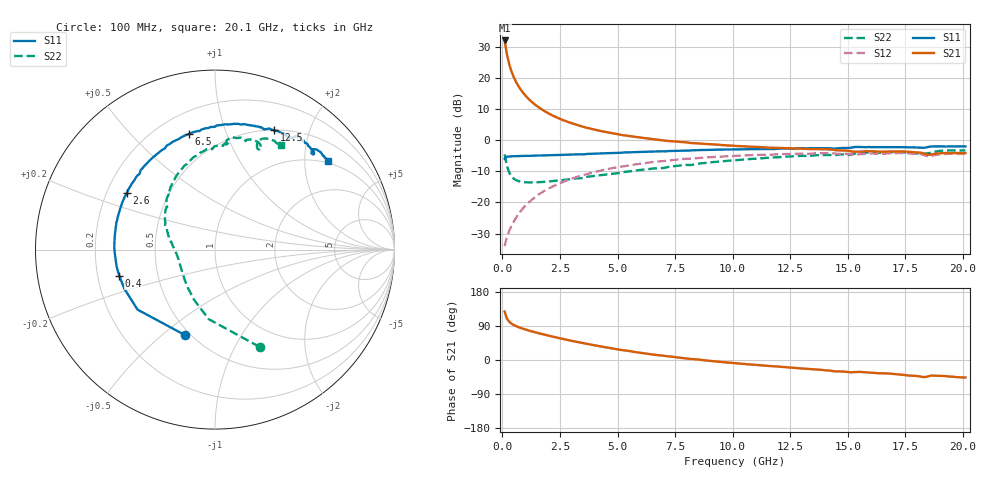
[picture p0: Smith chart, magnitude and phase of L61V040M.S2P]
!  Infineon Technologies AG
! BFR380L3 , PF131585-7, No.6, Th 09.10.01, soldered on pcb-board, measured with PP GSG850
!  Vce=1.0 V,  Ic=40.0 mA
! Common Emitter S-Parameters:  15. November 2001
#  GHz  S  MA  R  50
! f  S11  S21  S12  S22
! GHz  Mag  Ang  Mag  Ang  Mag  Ang  Mag  Ang
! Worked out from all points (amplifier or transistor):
!   201 points, 100 MHz to 20.1 GHz, reference 50 ohm
!   highest |S21| = 32.2 dB at 100 MHz (marker M1)
!   |S21| within 3 dB of that: start of sweep to 166.8 MHz
!   unconditionally stable (mu >= 1): 886.7 MHz to 4.66 GHz; 18.32 GHz to 18.54 GHz
!   at 3.4 GHz: K = 1.02, MAG = 7.1 dB, |S12| = -11.4 dB
!   at 10.1 GHz: K = 0.97, MSG = 1.6 dB, |S12| = -5.0 dB
!   at 20.1 GHz: K = 0.99, MSG = 0.1 dB, |S12| = -4.3 dB
!   S11 on the Smith chart (normalised r, x): 100 MHz: 0.47, -0.60; 400 MHz: 0.29, -0.12; 2.6 GHz: 0.28, +0.27; 6.5 GHz: 0.33, +0.75; 12.5 GHz: 0.50, +1.49; 20.1 GHz: 0.95, +2.58
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0.1  0.5047 -109.4  40.63 127.8  0.01979 59.6  0.5962 -65.4
0.2  0.546 -142.3  24.22 109.2  0.02799 54.9  0.389 -95.2
0.3  0.55 -156.6  16.86 101.1  0.0349 58.6  0.3032 -112.6
0.4  0.5532 -164.6  12.86 95.9  0.04201 61.6  0.2626 -124.7
0.5  0.5562 -170.0  10.37 92.2  0.04938 64.3  0.2413 -133.7
0.6  0.5566 -174.3  8.69 89.3  0.05715 65.7  0.2287 -140.5
0.7  0.5586 -177.6  7.484 86.7  0.06461 66.7  0.221 -146.0
0.8  0.561 179.3  6.567 84.5  0.0727 67.6  0.2162 -150.4
1  0.5624 174.5  5.288 80.5  0.08844 68.2  0.2116 -157.2
1.3  0.5655 168.5  4.101 75.2  0.1123 67.8  0.2105 -164.4
1.6  0.5697 162.9  3.362 70.3  0.136 66.6  0.2123 -169.6
2  0.5756 156.4  2.727 64.3  0.1668 64.4  0.2179 -175.1
2.6  0.5841 147.4  2.146 56.0  0.2119 60.5  0.2295 178.0
3.5  0.5955 135.0  1.657 44.5  0.2766 53.8  0.2474 169.5
4.9  0.6276 118.7  1.279 29.1  0.3642 43.2  0.2935 156.2
6.5  0.6618 102.6  1.051 14.7  0.4466 31.4  0.3511 141.8
6.8  0.6661 99.8  1.018 12.4  0.4592 29.0  0.3577 138.9
10.1  0.7187 76.2  0.8153 -8.3  0.5626 7.5  0.4794 114.1
12.5  0.7409 63.8  0.7443 -20.1  0.6071 -6.6  0.5513 96.8
13.5  0.747 59.4  0.7244 -24.4  0.6147 -12.1  0.5698 90.8
16.8  0.7781 47.5  0.662 -35.7  0.6162 -27.1  0.643 72.6
20.1  0.7983 38.2  0.626 -46.3  0.6095 -40.0  0.6907 58.0
